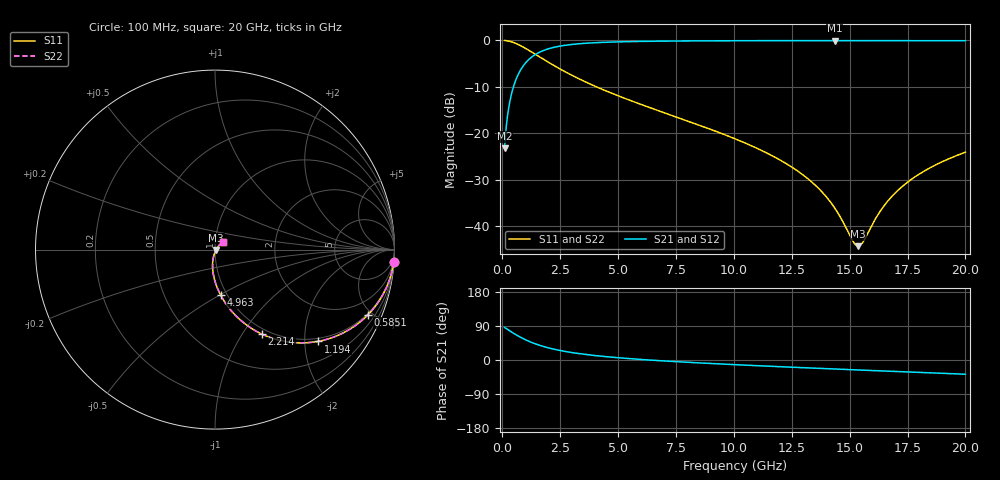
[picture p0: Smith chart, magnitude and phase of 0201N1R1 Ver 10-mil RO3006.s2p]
# GHz S MA R 50
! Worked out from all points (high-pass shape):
!   1601 points, 100 MHz to 20 GHz, reference 50 ohm
!   highest |S21| = -0.06 dB at 14.37 GHz (marker M1); lowest = -23.2 dB at 100 MHz (marker M2)
!   |S21| within 3 dB of the highest: 1.425 GHz to end of sweep
!   lowest |S11| = -44.3 dB at 15.37 GHz (marker M3), VSWR 1.01, Z = 50.5 - j0.276 ohm
!   |S11| at or under -10 dB: 4.064 GHz to end of sweep
!   |S22| runs from -44.3 to 0.0 dB; largest |S21 - S12| = 0
!   S11 on the Smith chart (normalised r, x): 100 MHz: 1, -28; 585.1 MHz: 0.92, -4.73; 1.194 GHz: 0.92, -2.31; 2.214 GHz: 0.93, -1.23; 4.963 GHz: 0.93, -0.51; 20 GHz: 1.09, +0.10
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0.1  0.9976 -4.1  0.06899 85.9  0.06899 85.9  0.9976 -4.1
0.323875  0.9757 -13.2  0.2186 76.8  0.2186 76.8  0.9757 -13.2
0.5850625  0.9265 -23.1  0.3753 66.9  0.3753 66.9  0.9265 -23.1
0.8586875  0.8586 -32.2  0.5112 57.7  0.5112 57.7  0.8586 -32.2
1.1945  0.7685 -41.7  0.638 48.1  0.638 48.1  0.7685 -41.7
1.692  0.6447 -52.6  0.7621 37.2  0.7621 37.2  0.6447 -52.6
2.214375  0.5388 -61.0  0.8397 28.8  0.8397 28.8  0.5388 -61.0
3.420812  0.3742 -73.5  0.924 16.0  0.924 16.0  0.3742 -73.5
4.963063  0.2554 -82.9  0.9629 6.2  0.9629 6.2  0.2554 -82.9
6.741625  0.1749 -90.2  0.9801 -1.6  0.9801 -1.6  0.1749 -90.2
10.05  0.08716 -99.0  0.9909 -12.3  0.9909 -12.3  0.08716 -99.0
11.99025  0.05157 -101.6  0.9929 -17.7  0.9929 -17.7  0.05157 -101.6
13.37081  0.02976 -100.2  0.9935 -21.3  0.9935 -21.3  0.02976 -100.2
14.36581  0.01555 -91.5  0.9936 -23.8  0.9936 -23.8  0.01555 -91.5
15.14937  0.006827 -53.5  0.9936 -25.8  0.9936 -25.8  0.006827 -53.5
15.37325  0.006083 -26.6  0.9935 -26.3  0.9935 -26.3  0.006083 -26.6
15.58469  0.00678 -1.4  0.9935 -26.8  0.9935 -26.8  0.00678 -1.4
16.19412  0.01292 32.8  0.9933 -28.3  0.9933 -28.3  0.01292 32.8
16.69162  0.01916 41.2  0.9931 -29.6  0.9931 -29.6  0.01916 41.2
17.30106  0.02707 45.2  0.9928 -31.0  0.9928 -31.0  0.02707 45.2
18.04731  0.03685 46.9  0.9923 -32.9  0.9923 -32.9  0.03685 46.9
20  0.06253 46.1  0.9907 -37.5  0.9907 -37.5  0.06253 46.1
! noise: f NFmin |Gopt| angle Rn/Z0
0.1  0.0009985  0.9605  0.9178  0.0057
2.301  0.005363  0.8265  4.64  0.006489
4.515  0.008287  0.7846  8.332  0.007862
6.729  0.01081  0.7579  12.04  0.008935
8.943  0.01311  0.7384  15.74  0.009845
11.14  0.01527  0.7233  19.4  0.01065
13.36  0.01734  0.7113  23.04  0.01138
15.57  0.01936  0.7016  26.65  0.01205
17.79  0.02133  0.6938  30.21  0.01269
20  0.02328  0.6875  33.73  0.01329
